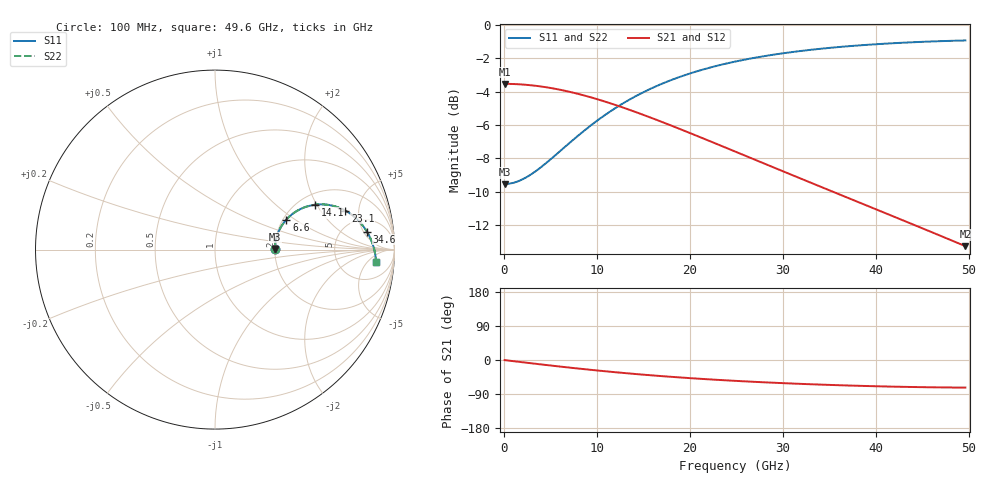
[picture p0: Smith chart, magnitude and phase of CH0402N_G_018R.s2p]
# GHz S RI R 18
! S-Parameters data
! Freq  reS11  imS11  reS21  imS21  reS12  imS12  reS22  imS22
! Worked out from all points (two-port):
!   100 points, 100 MHz to 49.6 GHz, reference 18 ohm
!   highest |S21| = -3.52 dB at 100 MHz (marker M1); lowest = -13.3 dB at 49.6 GHz (marker M2)
!   |S21| within 3 dB of the highest: start of sweep to 20.22 GHz
!   lowest |S11| = -9.5 dB at 100 MHz (marker M3), VSWR 2.00, Z = 36 + j0.23 ohm
!   |S11| at or under -10 dB: nowhere
!   |S22| runs from -9.5 to -0.9 dB; largest |S21 - S12| = 0
!   S11 on the Smith chart (normalised r, x): 100 MHz: 2.00, +0.01; 6.6 GHz: 2.08, +0.86; 14.1 GHz: 2.42, +1.93; 23.1 GHz: 3.48, +3.55; 34.6 GHz: 8, +6; 49.6 GHz: 13, -9
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0.1  0.3333 0.00284  0.6667 -0.00341  0.6667 -0.00341  0.3333 0.00284
1.1  0.3353 0.0312  0.6647 -0.0374  0.6647 -0.0374  0.3353 0.0312
2.6  0.3442 0.0726  0.6557 -0.0873  0.6557 -0.0873  0.3442 0.0726
3.6  0.3538 0.0988  0.646 -0.1192  0.646 -0.1192  0.3538 0.0988
4.6  0.3662 0.1236  0.6335 -0.1496  0.6335 -0.1496  0.3662 0.1236
6.6  0.3979 0.1674  0.6014 -0.2047  0.6014 -0.2047  0.3979 0.1674
8.6  0.4366 0.2022  0.5623 -0.2508  0.5623 -0.2508  0.4366 0.2022
9.6  0.4576 0.216  0.5409 -0.2703  0.5409 -0.2703  0.4576 0.216
11.1  0.4904 0.2323  0.5076 -0.295  0.5076 -0.295  0.4904 0.2323
12.6  0.5238 0.2435  0.4737 -0.3146  0.4737 -0.3146  0.5238 0.2435
14.1  0.5569 0.2499  0.4399 -0.3295  0.4399 -0.3295  0.5569 0.2499
16.6  0.6099 0.2514  0.3857 -0.3451  0.3857 -0.3451  0.6099 0.2514
19.6  0.6678 0.2412  0.3261 -0.3516  0.3261 -0.3516  0.6678 0.2412
23.1  0.7255 0.2174  0.266 -0.3475  0.266 -0.3475  0.7255 0.2174
25.1  0.7538 0.2  0.2362 -0.3412  0.2362 -0.3412  0.7538 0.2
29.1  0.8005 0.1601  0.186 -0.3236  0.186 -0.3236  0.8005 0.1601
33.1  0.8359 0.1165  0.1467 -0.3021  0.1467 -0.3021  0.8359 0.1165
34.6  0.8466 0.0997  0.1344 -0.2935  0.1344 -0.2935  0.8466 0.0997
38.1  0.867 0.0601  0.1101 -0.2731  0.1101 -0.2731  0.867 0.0601
41.6  0.8816 0.0207  0.0911 -0.2527  0.0911 -0.2527  0.8816 0.0207
45.6  0.8922 -0.0239  0.0751 -0.2297  0.0751 -0.2297  0.8922 -0.0239
49.6  0.8971 -0.0676  0.0643 -0.2074  0.0643 -0.2074  0.8971 -0.0676
